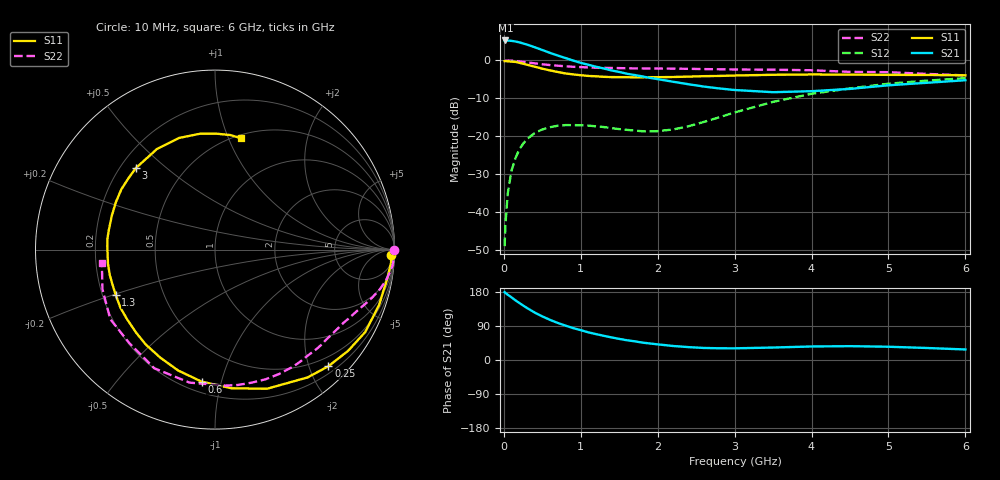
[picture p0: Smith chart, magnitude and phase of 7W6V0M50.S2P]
! Infineon Technologies  Discrete & RF Semiconductors
! BFS17W
! Si NPN RF Bipolar Junction Transistor in SOT323
! VCE = 6 V  IC = 0.5 mA
! Common Emitter S-Parameters:  August  1999
# GHz  S  MA  R  50
!  f  S11  S21  S12  S22
! GHz  MAG  ANG  MAG  ANG  MAG  ANG  MAG  ANG
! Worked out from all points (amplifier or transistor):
!   36 points, 10 MHz to 6 GHz, reference 50 ohm
!   highest |S21| = 5.3 dB at 20 MHz (marker M1)
!   |S21| within 3 dB of that: start of sweep to 564.6 MHz
!   unconditionally stable (mu >= 1): 1.243 GHz to end of sweep
!   at 250 MHz: K = 0.21, MSG = 13.2 dB, |S12| = -21.9 dB
!   at 1.4 GHz: K = 1.13, MAG = 5.4 dB, |S12| = -17.8 dB
!   at 6 GHz: K = 1.09, MAG = -2.1 dB, |S12| = -4.7 dB
!   S11 on the Smith chart (normalised r, x): 10 MHz: 30, -43; 250 MHz: 0.32, -2.33; 600 MHz: 0.27, -0.87; 1.3 GHz: 0.25, -0.20; 3 GHz: 0.26, +0.40; 6 GHz: 0.53, +1.11
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0.01  0.9787 -1.8  1.828 179.3  0.0036 88.1  0.9999 0.0
0.02  0.984 -4.1  1.831 177.1  0.0067 93.3  0.9839 -0.9
0.05  0.9734 -9.5  1.83 172.4  0.0176 85.7  0.9963 -2.5
0.1  0.9647 -18.7  1.806 165.3  0.0356 79.3  0.9933 -5.1
0.15  0.9546 -28.8  1.776 157.7  0.0515 72.9  0.9825 -7.4
0.25  0.9064 -45.8  1.673 143.9  0.08 63.0  0.9572 -11.7
0.3  0.8793 -54.1  1.617 137.4  0.0922 58.8  0.9443 -13.6
0.4  0.8277 -69.5  1.492 125.3  0.1106 50.5  0.9156 -17.0
0.5  0.7781 -83.2  1.371 115.1  0.1235 43.9  0.8899 -19.9
0.6  0.7393 -95.8  1.257 105.9  0.1323 38.8  0.8689 -22.4
0.8  0.6748 -116.8  1.077 90.7  0.141 31.4  0.8378 -27.3
1.1  0.6249 -141.7  0.876 72.9  0.1389 25.6  0.8089 -34.1
1.3  0.6081 -155.4  0.783 63.8  0.1329 25.0  0.7971 -39.1
1.6  0.6015 -172.4  0.668 52.1  0.1221 28.3  0.7876 -46.5
2.2  0.6052 161.8  0.524 37.0  0.1234 50.6  0.7796 -62.8
3  0.6331 134.1  0.408 30.8  0.2067 69.1  0.7599 -85.7
3.5  0.6472 119.9  0.382 32.9  0.285 67.9  0.7546 -100.8
4  0.6534 107.8  0.394 35.7  0.3637 62.2  0.7427 -117.1
4.5  0.651 97.4  0.422 36.5  0.4287 54.9  0.7066 -132.5
5  0.6459 89.3  0.471 35.0  0.4943 47.8  0.7005 -146.4
5.5  0.6438 82.4  0.508 31.7  0.5421 40.5  0.6648 -160.6
6  0.6371 76.9  0.549 27.8  0.5841 33.9  0.6352 -173.0
